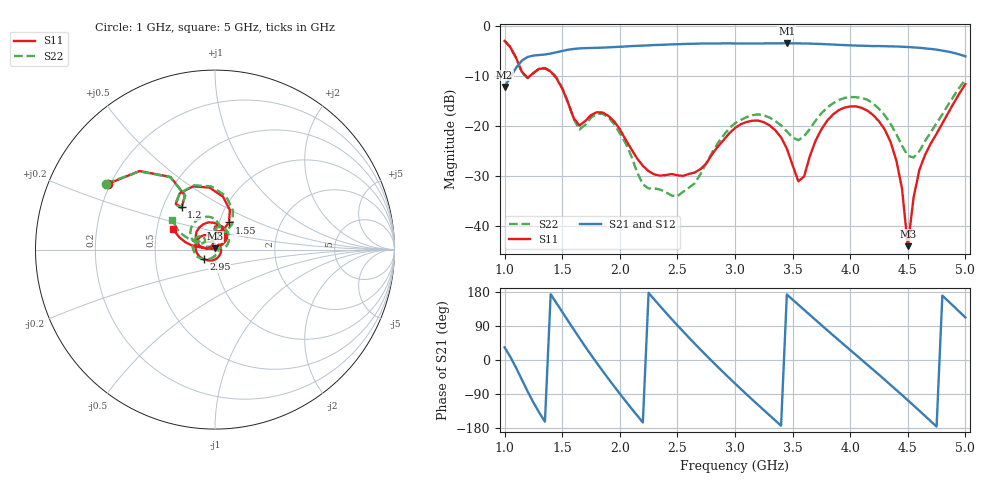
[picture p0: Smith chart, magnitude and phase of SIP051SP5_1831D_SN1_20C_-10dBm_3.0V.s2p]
# GHz  S  dB  R  50
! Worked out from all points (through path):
!   81 points, 1 GHz to 5 GHz, reference 50 ohm
!   highest |S21| = -3.55 dB at 3.45 GHz (marker M1); lowest = -12.2 dB at 1 GHz (marker M2)
!   lowest |S11| = -44.0 dB at 4.5 GHz (marker M3), VSWR 1.01, Z = 50 + j0.626 ohm
!   |S11| at or under -10 dB: 1.181 GHz to 1.224 GHz (42.62 MHz wide, 3.54 % of centre); 1.43 GHz to end of sweep
!   |S22| runs from -34.1 to -3.0 dB; largest |S21 - S12| = 0.0027
!   S11 on the Smith chart (normalised r, x): 1 GHz: 0.19, +0.27; 1.2 GHz: 0.62, +0.32; 1.55 GHz: 1.11, +0.35; 2.95 GHz: 0.88, -0.10; 5 GHz: 0.61, +0.15
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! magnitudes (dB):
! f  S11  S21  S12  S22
! 1 GHz  -3.1  -12.2  -12.2  -3.0
! 1.2 GHz  -10.5  -6.3  -6.3  -10.5
! 1.4 GHz  -9.2  -5.6  -5.6  -9.0
! 1.55 GHz  -15.4  -4.8  -4.8  -15.3
! 1.65 GHz  -20.0  -4.6  -4.6  -20.8
! 1.7 GHz  -19.1  -4.5  -4.5  -19.8
! 1.9 GHz  -18.0  -4.4  -4.4  -18.3
! 2.2 GHz  -28.0  -4.0  -4.0  -31.7
! 2.35 GHz  -30.0  -3.9  -3.9  -32.7
! 2.65 GHz  -29.4  -3.6  -3.6  -31.5
! 2.95 GHz  -21.5  -3.6  -3.6  -20.5
! 3 GHz  -20.5  -3.6  -3.6  -19.5
! 3.25 GHz  -19.3  -3.6  -3.6  -17.9
! 3.45 GHz  -24.6  -3.6  -3.6  -21.1
! 3.55 GHz  -31.1  -3.6  -3.6  -22.9
! 3.7 GHz  -23.0  -3.7  -3.7  -19.0
! 4.05 GHz  -16.1  -4.0  -4.0  -14.3
! 4.35 GHz  -23.2  -4.2  -4.2  -19.6
! 4.45 GHz  -32.6  -4.2  -4.2  -24.0
! 4.5 GHz  -44.0  -4.3  -4.3  -26.0
! 4.6 GHz  -28.9  -4.4  -4.5  -25.1
! 5 GHz  -11.7  -6.2  -6.2  -10.8
